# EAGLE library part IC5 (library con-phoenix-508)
PHOENIX
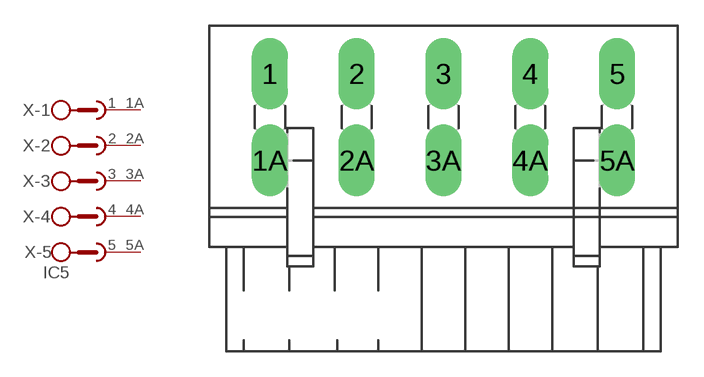
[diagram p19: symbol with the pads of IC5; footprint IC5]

Designator prefix X; gates -1=SKB2 -2=SKB2 -3=SKB2 -4=SKB2 -5=SKB2V

## IC5 (OC_FARNELL: unknown; OC_NEWARK: unknown)  [IC5]
1  -1:1  pas
1A  -1:2  pas
2  -2:1  pas
2A  -2:2  pas
3  -3:1  pas
3A  -3:2  pas
4  -4:1  pas
4A  -4:2  pas
5  -5:1  pas
5A  -5:2  pas

## Footprint IC5 (pad centres in mm)
PHOENIX
drill 1.397 long: 1 -10.16,2.54; 1A -10.16,-2.54; 2 -5.08,2.54; 2A -5.08,-2.54; 3 0,2.54; 3A 0,-2.54; 4 5.08,2.54; 4A 5.08,-2.54; 5 10.16,2.54; 5A 10.16,-2.54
